PROGRAM MAIN
VAR
	AODB			: ARRAY[0..49] OF ST_IEC870_5_101AODBEntry; (* Application object data base (data points)*)
	hTable			: T_HAODBTable;(* Application object database handle *)
	fbClient		: FB_IEC870_5_104Master;(* IEC 60870-5-104 master function block instance *)
	fbHandler		: FB_IEC870_5_101TableEventHandler;

	nCAA			: UDINT := 7;(* Common ASDU address of remote (slave) station *)

	inputs AT%I*	: ARRAY[0..2999] OF BYTE;
	outputs AT%Q*	: ARRAY[0..2999] OF BYTE;
	memory AT%M*	: ST_MemoryData;
	data 			: ARRAY[0..2999] OF BYTE;

	bEnable			: BOOL := TRUE;(* Enable/disable communication *)
	bSendCmd		: BOOL := FALSE;(* If TRUE => Enable sending of commands *)
	bTrigSc11		: BOOL := FALSE;(* Rising edge at this variable triggers single command execution, ioa := 11 *)
	bTrigDc21		: BOOL := FALSE;(* Rising edge at this variable triggers double command execution, ioa := 21 *)
	bTrigRc31		: BOOL := FALSE;(* Rising edge at this variable triggers regulating step command execution, ioa := 31 *)
	bTrigBo41		: BOOL := FALSE;(* Rising edge at this variable triggers setpoint command execution, ioa := 41 *)
	bTrigSp51		: BOOL := FALSE;(* Rising edge at this variable triggers setpoint command execution, ioa := 51 *)
	bTrigSp61		: BOOL := FALSE;(* Rising edge at this variable triggers setpoint command execution, ioa := 61 *)
	bTrigSp71		: BOOL := FALSE;(* Rising edge at this variable triggers setpoint command execution, ioa := 71 *)

	bInit			: BOOL := TRUE;
	fbTimer			: TON := ( PT := T#10S );
	fbCloseAll		: FB_SocketCloseAll;
	nInitErr		: UDINT;
	nTrigErr		: UDINT;

END_VAR

fbCloseAll( bExecute := bInit );
IF fbCloseAll.bBusy AND NOT bInit THEN
	RETURN;
END_IF

IF bInit THEN
	bInit := FALSE;

	(* Configure protocol parameter *)
	fbClient.protPara.sRemoteHost 			:= '127.0.0.1';(* Remote (server) address. String containing an (Ipv4) Internet Protocol dotted address. *)
	fbClient.protPara.nRemotePort 			:= 2404;(* Remote (server) Internet Protocol (IP) port. Default = 2404 *)
	fbClient.protPara.t0					:= T#30S;(* MASTER only: Connection establishment, Default = 30s *)
	fbClient.protPara.t1 					:= T#15S;(* Response Timeout (STARTDTAct, STOPDTAct, TESTFRAct only, Default = 15s ) *)
	fbClient.protPara.t2 					:= T#10S;(* Send ACK in case of no data frames, Default = 10s *)
	fbClient.protPara.t3 					:= T#20S;(* Time for sending test frames, Default = 20s *)
	fbClient.protPara.iK 					:= 12;(* Max. difference RSN to send ACK , Default = 12 *)
	fbClient.protPara.iW 					:= 8;(* Latest ACK after receiving I-frames, Default = 8 *)
	fbClient.protPara.bThrottleMode 		:= TRUE;(* If set reduces the number of polling socket read requests *)
	fbClient.protPara.bPackFrames			:= TRUE;(* Binds more than one APDU frame to one big TCP/IP frame *)

	(* Configure system parameter *)
	fbClient.sysPara.asduAddr 				:= nCAA;
	fbClient.sysPara.asduFmt.eCOTSize 		:= eIEC870_COT_TwoOctets;(* Cause of transfer octet size *)
	fbClient.sysPara.asduFmt.eAsduAddrSize 	:= eIEC870_AsduAddr_TwoOctets;(* Common ASDU address octet size *)
	fbClient.sysPara.asduFmt.eObjAddrSize 	:= eIEC870_ObjAddr_ThreeOctets;(* Object address octet size *)
	fbClient.sysPara.dbgMode 				:= IEC870_DEBUGMODE_DEVSTATE OR IEC870_DEBUGMODE_LINKERROR(* OR IEC870_DEBUGMODE_LINKLAYER OR IEC870_DEBUGMODE_ASDU *);

	(* Configure data aquisition parameter (clock synchronisation, test commands, general interrogation, counter interrogation...) *)
	fbClient.acqPara.arrInitSeq[0] 			:= eIEC870_ISTEP_UNUSED;(* Disable test command at initialization *)

	fbClient.acqPara.clockSync.tPollCycle	:= T#60S; 
	fbClient.acqPara.clockSync.bEnable		:= TRUE;(* Enable cyclic clock synchronisation *)

	fbClient.acqPara.testCmd.tPollCycle		:= T#60S; 
	fbClient.acqPara.testCmd.bEnable		:= TRUE;(* Enable cylclic test command *)

	fbClient.acqPara.arrGenro[0].eQOI 		:= eIEC870_QOI_INROGEN;
	fbClient.acqPara.arrGenro[0].tPollCycle := T#60S;
	fbClient.acqPara.arrGenro[0].bEnable 	:= TRUE;(* Enable general interrogation *)
	
	fbClient.acqPara.arrCoro[0].eFRZ		:= eIEC870_FRZ_READ; 
	fbClient.acqPara.arrCoro[0].eRQT		:= eIEC870_RQT_REQCOGEN;
	fbClient.acqPara.arrCoro[0].tPollCycle	:= T#60S;
	fbClient.acqPara.arrCoro[0].bEnable 	:= FALSE;(* Disable counter interrogation => Use MODE A: local freeze with spontaneous transfer *)
//	fbClient.acqPara.arrCoro[0].bEnable 	:= TRUE;(* Enable counter interrogation => Use Mode B: Local freeze with counter interrogation *)
	
	nInitErr := F_iecCreateTableHnd( ADR( AODB ), SIZEOF( AODB ), hTable );
	
	(* Monitored Single points *)
	nInitErr := F_iecAddTableEntry( M_SP_NA_1, nCAA, 100, IEC870_GRP_INROGEN, 0, MAP_AREA_MEMORY, ADR( memory.eSPI_100_msg ) - ADR( memory ), 0, 0, hTable );
	nInitErr := F_iecAddTableEntry( M_SP_NA_1, nCAA, 101, IEC870_GRP_INROGEN, 0, MAP_AREA_MEMORY, ADR( memory.eSPI_101_msg ) - ADR( memory ), 0, 0, hTable );
	nInitErr := F_iecAddTableEntry( M_SP_TB_1, nCAA, 102, IEC870_GRP_INROGEN, 0, MAP_AREA_MEMORY, ADR( memory.eSPI_102_msg ) - ADR( memory ), 0, 0, hTable );
	(* Double points*)
	nInitErr := F_iecAddTableEntry( M_DP_NA_1, nCAA, 200, IEC870_GRP_INROGEN, 0, MAP_AREA_MEMORY, ADR( memory.eDPI_200_msg ) - ADR( memory ), 0, 0, hTable );
	nInitErr := F_iecAddTableEntry( M_DP_NA_1, nCAA, 201, IEC870_GRP_INROGEN, 0, MAP_AREA_MEMORY, ADR( memory.eDPI_201_msg ) - ADR( memory ), 0, 0, hTable );
	nInitErr := F_iecAddTableEntry( M_DP_TB_1, nCAA, 202, IEC870_GRP_INROGEN, 0, MAP_AREA_MEMORY, ADR( memory.eDPI_202_msg ) - ADR( memory ), 0, 0, hTable );
	(* Regulating step values *)
	nInitErr := F_iecAddTableEntry( M_ST_NA_1, nCAA, 300, IEC870_GRP_INROGEN, 0, MAP_AREA_MEMORY, ADR( memory.nVTI_300_msg ) - ADR( memory ), 0, 0, hTable );
	nInitErr := F_iecAddTableEntry( M_ST_NA_1, nCAA, 301, IEC870_GRP_INROGEN, 0, MAP_AREA_MEMORY, ADR( memory.nVTI_301_msg ) - ADR( memory ), 0, 0, hTable );
	nInitErr := F_iecAddTableEntry( M_ST_TB_1, nCAA, 302, IEC870_GRP_INROGEN, 0, MAP_AREA_MEMORY, ADR( memory.nVTI_302_msg ) - ADR( memory ), 0, 0, hTable );
	(* 32 bit strings *)
	nInitErr := F_iecAddTableEntry( M_BO_NA_1, nCAA, 400, IEC870_GRP_INROGEN, 0, MAP_AREA_MEMORY, ADR( memory.nBSI_400_msg ) - ADR( memory ), 0, 0, hTable );
	nInitErr := F_iecAddTableEntry( M_BO_NA_1, nCAA, 401, IEC870_GRP_INROGEN, 0, MAP_AREA_MEMORY, ADR( memory.nBSI_401_msg ) - ADR( memory ), 0, 0, hTable );
	nInitErr := F_iecAddTableEntry( M_BO_TB_1, nCAA, 402, IEC870_GRP_INROGEN, 0, MAP_AREA_MEMORY, ADR( memory.nBSI_402_msg ) - ADR( memory ), 0, 0, hTable );
	(* Measured values, normalized values *)
	nInitErr := F_iecAddTableEntry( M_ME_NA_1, nCAA, 500, IEC870_GRP_INROGEN, 0, MAP_AREA_MEMORY, ADR( memory.nNVA_500_msg ) - ADR( memory ), 0, 0, hTable );
	nInitErr := F_iecAddTableEntry( M_ME_NA_1, nCAA, 501, IEC870_GRP_INROGEN, 0, MAP_AREA_MEMORY, ADR( memory.nNVA_501_msg ) - ADR( memory ), 0, 0, hTable );
	nInitErr := F_iecAddTableEntry( M_ME_TD_1, nCAA, 502, IEC870_GRP_INROGEN, 0, MAP_AREA_MEMORY, ADR( memory.nNVA_502_msg ) - ADR( memory ), 0, 0, hTable );
	(* Mesured values, scaled values *)
	nInitErr := F_iecAddTableEntry( M_ME_NB_1, nCAA, 600, IEC870_GRP_INROGEN, 0, MAP_AREA_MEMORY, ADR( memory.nSVA_600_msg ) - ADR( memory ), 0, 0, hTable );
	nInitErr := F_iecAddTableEntry( M_ME_NB_1, nCAA, 601, IEC870_GRP_INROGEN, 0, MAP_AREA_MEMORY, ADR( memory.nSVA_601_msg ) - ADR( memory ), 0, 0, hTable );
	nInitErr := F_iecAddTableEntry( M_ME_TE_1, nCAA, 602, IEC870_GRP_INROGEN, 0, MAP_AREA_MEMORY, ADR( memory.nSVA_602_msg ) - ADR( memory ), 0, 0, hTable );
	(* Measured values , short floating point values *)
	nInitErr := F_iecAddTableEntry( M_ME_NC_1, nCAA, 700, IEC870_GRP_INROGEN, 0, MAP_AREA_MEMORY, ADR( memory.fR32_700_msg ) - ADR( memory ), 0, 0, hTable );
	nInitErr := F_iecAddTableEntry( M_ME_NC_1, nCAA, 701, IEC870_GRP_INROGEN, 0, MAP_AREA_MEMORY, ADR( memory.fR32_701_msg ) - ADR( memory ), 0, 0, hTable );
	nInitErr := F_iecAddTableEntry( M_ME_TF_1, nCAA, 702, IEC870_GRP_INROGEN, 0, MAP_AREA_MEMORY, ADR( memory.fR32_702_msg ) - ADR( memory ), 0, 0, hTable );
	(* Integrated totals *)
	nInitErr := F_iecAddTableEntry( M_IT_NA_1, nCAA, 800, IEC870_GRP_REQCOGEN, 0, MAP_AREA_MEMORY, ADR( memory.nBCR_800_msg ) - ADR( memory ), 0, 0, hTable );
	nInitErr := F_iecAddTableEntry( M_IT_NA_1, nCAA, 801, IEC870_GRP_REQCOGEN, 0, MAP_AREA_MEMORY, ADR( memory.nBCR_801_msg ) - ADR( memory ), 0, 0, hTable );
	nInitErr := F_iecAddTableEntry( M_IT_TB_1, nCAA, 802, IEC870_GRP_REQCOGEN, 0, MAP_AREA_MEMORY, ADR( memory.nBCR_802_msg ) - ADR( memory ), 0, 0, hTable );

	(* Controlled Single commands *)
	nInitErr := F_iecAddTableEntry( C_SC_NA_1, nCAA, 10, 0, 0, MAP_AREA_MEMORY, ADR( memory.eSCS_10_cmd ) - ADR( memory ), 0, 0, hTable );
	nInitErr := F_iecAddTableEntry( C_SC_NA_1, nCAA, 11, IEC870_GRP_SPONTOFF, 0, MAP_AREA_MEMORY, ADR( memory.eSCS_11_cmd ) - ADR( memory ), 0, 0, hTable );
	nInitErr := F_iecAddTableEntry( C_SC_TA_1, nCAA, 12, 0, 0, MAP_AREA_MEMORY, ADR( memory.eSCS_12_cmd ) - ADR( memory ), 0, 0, hTable );
	(* Double commands *)
	nInitErr := F_iecAddTableEntry( C_DC_NA_1, nCAA, 20, 0, 0, MAP_AREA_MEMORY, ADR( memory.eDCS_20_cmd ) - ADR( memory ), 0, 0, hTable );
	nInitErr := F_iecAddTableEntry( C_DC_NA_1, nCAA, 21, IEC870_GRP_SPONTOFF, 0, MAP_AREA_MEMORY, ADR( memory.eDCS_21_cmd ) - ADR( memory ), 0, 0, hTable );
	nInitErr := F_iecAddTableEntry( C_DC_TA_1, nCAA, 22, 0, 0, MAP_AREA_MEMORY, ADR( memory.eDCS_22_cmd ) - ADR( memory ), 0, 0, hTable );
	(* Regulating step commands *)
	nInitErr := F_iecAddTableEntry( C_RC_NA_1, nCAA, 30, 0, 0, MAP_AREA_MEMORY, ADR( memory.eRCS_30_cmd ) - ADR( memory ), 0, 0, hTable );
	nInitErr := F_iecAddTableEntry( C_RC_NA_1, nCAA, 31, IEC870_GRP_SPONTOFF, 0, MAP_AREA_MEMORY, ADR( memory.eRCS_31_cmd ) - ADR( memory ), 0, 0, hTable );
	nInitErr := F_iecAddTableEntry( C_RC_TA_1, nCAA, 32, 0, 0, MAP_AREA_MEMORY, ADR( memory.eRCS_32_cmd ) - ADR( memory ), 0, 0, hTable );
	(* Bistring commands*)
	nInitErr := F_iecAddTableEntry( C_BO_NA_1, nCAA, 40, 0, 0, MAP_AREA_MEMORY, ADR( memory.nBSI_40_cmd ) - ADR( memory ), 0, 0, hTable );
	nInitErr := F_iecAddTableEntry( C_BO_NA_1, nCAA, 41, IEC870_GRP_SPONTOFF, 0, MAP_AREA_MEMORY, ADR( memory.nBSI_41_cmd ) - ADR( memory ), 0, 0, hTable );
	nInitErr := F_iecAddTableEntry( C_BO_TA_1, nCAA, 42, 0, 0, MAP_AREA_MEMORY, ADR( memory.nBSI_42_cmd ) - ADR( memory ), 0, 0, hTable );
	(* Set-point Command, normalised value *)
	nInitErr := F_iecAddTableEntry( C_SE_NA_1, nCAA, 50, 0, 0, MAP_AREA_MEMORY, ADR( memory.nNVA_50_cmd ) - ADR( memory ), 0, 0, hTable );
	nInitErr := F_iecAddTableEntry( C_SE_NA_1, nCAA, 51, IEC870_GRP_SPONTOFF, 0, MAP_AREA_MEMORY, ADR( memory.nNVA_51_cmd ) - ADR( memory ), 0, 0, hTable );
	nInitErr := F_iecAddTableEntry( C_SE_TA_1, nCAA, 52, 0, 0, MAP_AREA_MEMORY, ADR( memory.nNVA_52_cmd ) - ADR( memory ), 0, 0, hTable );
	(* Set-point Command, scalled value *)
	nInitErr := F_iecAddTableEntry( C_SE_NB_1, nCAA, 60, 0, 0, MAP_AREA_MEMORY, ADR( memory.nSVA_60_cmd ) - ADR( memory ), 0, 0, hTable );
	nInitErr := F_iecAddTableEntry( C_SE_NB_1, nCAA, 61, IEC870_GRP_SPONTOFF, 0, MAP_AREA_MEMORY, ADR( memory.nSVA_61_cmd ) - ADR( memory ), 0, 0, hTable );
	nInitErr := F_iecAddTableEntry( C_SE_TB_1, nCAA, 62, 0, 0, MAP_AREA_MEMORY, ADR( memory.nSVA_62_cmd ) - ADR( memory ), 0, 0, hTable );
	(* Set-point Command, short floating point value *)
	nInitErr := F_iecAddTableEntry( C_SE_NC_1, nCAA, 70, 0, 0, MAP_AREA_MEMORY, ADR( memory.fR32_70_cmd ) - ADR( memory ), 0, 0, hTable );
	nInitErr := F_iecAddTableEntry( C_SE_NC_1, nCAA, 71, IEC870_GRP_SPONTOFF, 0, MAP_AREA_MEMORY, ADR( memory.fR32_71_cmd ) - ADR( memory ), 0, 0, hTable );
	nInitErr := F_iecAddTableEntry( C_SE_TC_1, nCAA, 72, 0, 0, MAP_AREA_MEMORY, ADR( memory.fR32_72_cmd ) - ADR( memory ), 0, 0, hTable );
	
ELSE
	(* Execute IEC master function block *)
	fbClient(	pAOEntries	:= ADR( AODB ),
				cbAOEntries := SIZEOF( AODB ),
				pInputs 	:= ADR( inputs ),
				cbInputs 	:= SIZEOF( inputs ),
				pOutputs 	:= ADR( outputs ),
				cbOutputs 	:= SIZEOF( outputs ),
				pMemory 	:= ADR( memory ),
				cbMemory 	:= SIZEOF( memory ),
				pData 		:= ADR( data ),
				cbData 		:= SIZEOF( data ),
				hTable 		:= hTable,
				bEnable 	:= bEnable );
	
	
	(* Log errors *)
	REPEAT
		fbClient.system.device.errors.RemoveError( );
		IF fbClient.system.device.errors.bOk THEN
			ADSLOGSTR( ADSLOG_MSGTYPE_ERROR OR ADSLOG_MSGTYPE_LOG, 'IEC60870-5-104 master communication error: 0x%s',
						DWORD_TO_HEXSTR( fbClient.system.device.errors.getError.nErrId, 8, FALSE) );
		END_IF
	UNTIL NOT fbClient.system.device.errors.bOk
	END_REPEAT

	(* Log events *)
	REPEAT
		fbHandler.RemoveOnChangeEvent( hTable := hTable );
		IF fbHandler.bOk THEN
			ADSLOGSTR( ADSLOG_MSGTYPE_HINT OR ADSLOG_MSGTYPE_LOG, 'IEC60870-5-104 master RemoveOnChangeEvent(), IOA: %s',
						DWORD_TO_STRING( fbHandler.getObj.info.objAddr ) );
		END_IF
	UNTIL NOT fbHandler.bOk
	END_REPEAT


	REPEAT
		fbHandler.RemoveOnCreateEvent( hTable := hTable );
		IF fbHandler.bOk THEN
			ADSLOGSTR( ADSLOG_MSGTYPE_HINT OR ADSLOG_MSGTYPE_LOG, 'IEC60870-5-104 master RemoveOnCreateEvent(), IOA: %s',
						DWORD_TO_STRING( fbHandler.getObj.info.objAddr ) );
		END_IF
	UNTIL NOT fbHandler.bOk
	END_REPEAT

END_IF


(* Simple command simulation *)
fbTimer( IN := bSendCmd ); 
IF fbTimer.Q THEN(* => send command *)
	fbTimer( IN := FALSE );
	fbTimer( IN := bSendCmd );
 
	(* Toggle single commands ON<->OFF *)
	memory.eSCS_10_cmd := SEL( memory.eSCS_10_cmd = eIEC870_SCS_OFF, eIEC870_SCS_OFF, eIEC870_SCS_ON );
	memory.eSCS_12_cmd := SEL( memory.eSCS_12_cmd = eIEC870_SCS_OFF, eIEC870_SCS_OFF, eIEC870_SCS_ON );

	(* Toggle double commands ON<->OFF *)
	memory.eDCS_20_cmd := SEL( memory.eDCS_20_cmd = eIEC870_DCS_OFF, eIEC870_DCS_OFF, eIEC870_DCS_ON );
	memory.eDCS_22_cmd := SEL( memory.eDCS_22_cmd = eIEC870_DCS_OFF, eIEC870_DCS_OFF, eIEC870_DCS_ON );

	(* Toggle regulating step commands UP<->DOWN *)
	memory.eRCS_30_cmd := SEL( memory.eRCS_30_cmd = eIEC870_RCS_INCREMENT, eIEC870_RCS_INCREMENT, eIEC870_RCS_DECREMENT );
	memory.eRCS_32_cmd := SEL( memory.eRCS_32_cmd = eIEC870_RCS_INCREMENT, eIEC870_RCS_INCREMENT, eIEC870_RCS_DECREMENT );
	
	(* Modify bitstring command values *)
	memory.nBSI_40_cmd := memory.nBSI_40_cmd + 1;
	memory.nBSI_42_cmd := memory.nBSI_42_cmd + 3;
	
	(* Modify setpoint values  *)
	memory.nNVA_50_cmd := memory.nNVA_50_cmd + 4;
	memory.nNVA_52_cmd := memory.nNVA_52_cmd + 6;

	memory.nSVA_60_cmd := memory.nSVA_60_cmd + 7;
	memory.nSVA_62_cmd := memory.nSVA_62_cmd + 9;

	memory.fR32_70_cmd := memory.fR32_70_cmd + 1.1;
	memory.fR32_72_cmd := memory.fR32_72_cmd + 1.3;
	
END_IF

IF bTrigSc11 THEN(* Trigger single command *)
	bTrigSc11 := FALSE;
	memory.eSCS_11_cmd := SEL( memory.eSCS_11_cmd = eIEC870_SCS_OFF, eIEC870_SCS_OFF, eIEC870_SCS_ON );
	nTrigErr := F_iecTriggerScDcRcCmdTableEntry( C_SC_NA_1, nCAA, 11, FALSE, eIEC870_QU_UNSPECIFIED, FALSE, hTable );
	IF nTrigErr <> 0 THEN
		ADSLOGSTR( ADSLOG_MSGTYPE_ERROR OR ADSLOG_MSGTYPE_LOG, 'F_iecTriggerScDcRcCmdTableEntry(C_SC_NA_1) error:%s', DWORD_TO_HEXSTR( nTrigErr, 8, FALSE) );
	END_IF	
END_IF

IF bTrigDc21 THEN(* Trigger double command *)
	bTrigDc21 := FALSE;
	memory.eDCS_21_cmd := SEL( memory.eDCS_21_cmd = eIEC870_DCS_OFF, eIEC870_DCS_OFF, eIEC870_DCS_ON );
	nTrigErr := F_iecTriggerScDcRcCmdTableEntry( C_DC_NA_1, nCAA, 21, FALSE, eIEC870_QU_UNSPECIFIED, FALSE, hTable );
	IF nTrigErr <> 0 THEN
		ADSLOGSTR( ADSLOG_MSGTYPE_ERROR OR ADSLOG_MSGTYPE_LOG, 'F_iecTriggerScDcRcCmdTableEntry(C_DC_NA_1) error:%s', DWORD_TO_HEXSTR( nTrigErr, 8, FALSE) );
	END_IF	
END_IF

IF bTrigRc31 THEN(* Trigger regulating step command *)
	bTrigRc31 := FALSE;
	memory.eRCS_31_cmd := SEL( memory.eRCS_31_cmd = eIEC870_RCS_INCREMENT, eIEC870_RCS_INCREMENT, eIEC870_RCS_DECREMENT );
	nTrigErr := F_iecTriggerScDcRcCmdTableEntry( C_RC_NA_1, nCAA, 31, FALSE, eIEC870_QU_UNSPECIFIED, FALSE, hTable );
	IF nTrigErr <> 0 THEN
		ADSLOGSTR( ADSLOG_MSGTYPE_ERROR OR ADSLOG_MSGTYPE_LOG, 'F_iecTriggerScDcRcCmdTableEntry(C_RC_NA_1) error:%s', DWORD_TO_HEXSTR( nTrigErr, 8, FALSE) );
	END_IF	
END_IF

IF bTrigBo41 THEN(* Trigger bitstring command *)
	bTrigBo41 := FALSE;
	memory.nBSI_41_cmd := memory.nBSI_41_cmd + 2;
	nTrigErr := F_iecTriggerScDcRcCmdTableEntry( C_BO_NA_1, nCAA, 41, FALSE, 0, FALSE, hTable );
	IF nTrigErr <> 0 THEN
		ADSLOGSTR( ADSLOG_MSGTYPE_ERROR OR ADSLOG_MSGTYPE_LOG, 'F_iecTriggerScDcRcCmdTableEntry(C_BO_NA_1) error:%s', DWORD_TO_HEXSTR( nTrigErr, 8, FALSE) );
	END_IF	
END_IF

IF bTrigSp51 THEN(* Trigger setpoint command, normalized value *)
	bTrigSp51 := FALSE;
	memory.nNVA_51_cmd := memory.nNVA_51_cmd + 5;
	nTrigErr := F_iecTriggerSetpointCmdTableEntry( C_SE_NA_1, nCAA, 51, FALSE, eIEC870_QL_DEFAULT, FALSE, hTable );
	IF nTrigErr <> 0 THEN
		ADSLOGSTR( ADSLOG_MSGTYPE_ERROR OR ADSLOG_MSGTYPE_LOG, 'F_iecTriggerSetpointCmdTableEntry(C_SE_NA_1) error:%s', DWORD_TO_HEXSTR( nTrigErr, 8, FALSE) );
	END_IF	
END_IF

IF bTrigSp61 THEN(* Trigger setpoint command, scaled value *)
	bTrigSp61 := FALSE;
	memory.nSVA_61_cmd := memory.nSVA_61_cmd + 8;
	nTrigErr := F_iecTriggerSetpointCmdTableEntry( C_SE_NB_1, nCAA, 61, FALSE, eIEC870_QL_DEFAULT, FALSE, hTable );
	IF nTrigErr <> 0 THEN
		ADSLOGSTR( ADSLOG_MSGTYPE_ERROR OR ADSLOG_MSGTYPE_LOG, 'F_iecTriggerSetpointCmdTableEntry(C_SE_NB_1) error:%s', DWORD_TO_HEXSTR( nTrigErr, 8, FALSE) );
	END_IF	
END_IF

IF bTrigSp71 THEN(* Trigger setpoint command, short floating point value *)
	bTrigSp71 := FALSE;
	memory.fR32_71_cmd := memory.fR32_71_cmd + 1.2;
	nTrigErr := F_iecTriggerSetpointCmdTableEntry( C_SE_NC_1, nCAA, 71, FALSE, eIEC870_QL_DEFAULT, FALSE, hTable );
	IF nTrigErr <> 0 THEN
		ADSLOGSTR( ADSLOG_MSGTYPE_ERROR OR ADSLOG_MSGTYPE_LOG, 'F_iecTriggerSetpointCmdTableEntry(C_SE_NC_1) error:%s', DWORD_TO_HEXSTR( nTrigErr, 8, FALSE) );
	END_IF	
END_IF

END_PROGRAM
